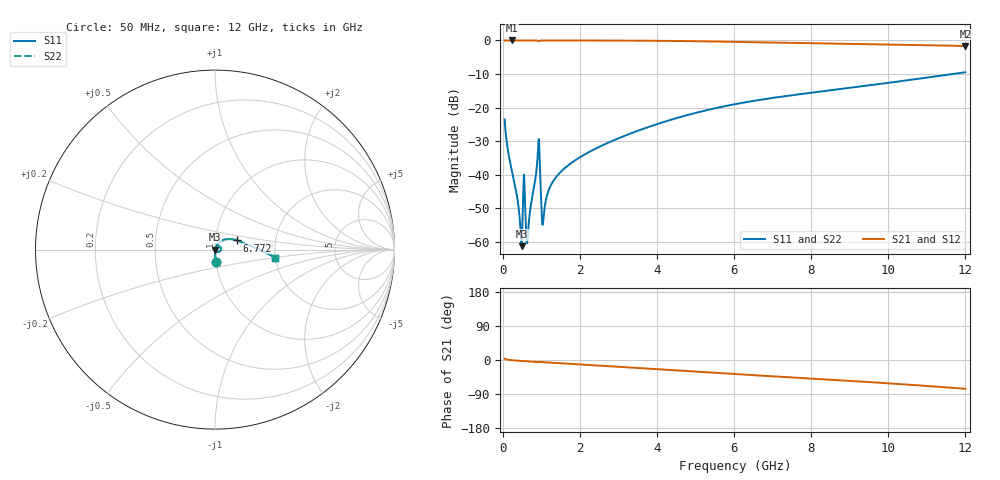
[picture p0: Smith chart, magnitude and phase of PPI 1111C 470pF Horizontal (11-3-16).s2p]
# MHz S MA R 50
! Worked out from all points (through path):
!   1601 points, 50 MHz to 12 GHz, reference 50 ohm
!   highest |S21| = 0.00 dB at 244.2 MHz (marker M1); lowest = -1.7 dB at 12 GHz (marker M2)
!   group delay of S21, straight-line fit = 17.5 ps
!   lowest |S11| = -61.3 dB at 490.7 MHz (marker M3), VSWR 1.00, Z = 50.1 - j0.00423 ohm
!   |S11| at or under -10 dB: start of sweep to 11.67 GHz
!   |S22| runs from -61.3 to -9.5 dB; largest |S21 - S12| = 0
!   S11 on the Smith chart (normalised r, x): 50 MHz: 1.00, -0.13; 6.772 GHz: 1.27, +0.13; 12 GHz: 1.98, -0.20
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50  0.06664 -86.2  0.9975 3.6  0.9975 3.6  0.06664 -86.2
244.1875  0.01111 -88.4  0.9995 -0.7  0.9995 -0.7  0.01111 -88.4
371.1562  0.004795 -85.4  0.9994 -1.7  0.9994 -1.7  0.004795 -85.4
445.8438  0.002067 -74.4  0.9993 -2.3  0.9993 -2.3  0.002067 -74.4
468.25  0.001279 -58.9  0.9993 -2.4  0.9993 -2.4  0.001279 -58.9
490.6562  0.0008631 -2.8  0.9991 -2.6  0.9991 -2.6  0.0008631 -2.8
565.3438  0.006683 -45.5  0.995 -2.7  0.995 -2.7  0.006683 -45.5
632.5625  0.0009554 9.8  0.999 -3.4  0.999 -3.4  0.0009554 9.8
662.4375  0.001539 52.9  0.9991 -3.6  0.9991 -3.6  0.001539 52.9
908.9062  0.01957 60.9  0.9921 -5.9  0.9921 -5.9  0.01957 60.9
946.25  0.02812 -24.0  0.9734 -4.5  0.9734 -4.5  0.02812 -24.0
1020.938  0.002078 -19.5  0.9979 -5.4  0.9979 -5.4  0.002078 -19.5
1058.281  0.002292 45.7  0.9985 -5.7  0.9985 -5.7  0.002292 45.7
1177.781  0.005566 72.6  0.9989 -6.6  0.9989 -6.6  0.005566 72.6
1334.625  0.008427 75.5  0.9989 -7.6  0.9989 -7.6  0.008427 75.5
2044.156  0.01882 73.3  0.9981 -11.9  0.9981 -11.9  0.01882 73.3
4038.312  0.0576 55.1  0.9876 -24.4  0.9876 -24.4  0.0576 55.1
6025  0.1124 30.8  0.9519 -37.1  0.9519 -37.1  0.1124 30.8
6771.875  0.1331 22.6  0.9346 -41.6  0.9346 -41.6  0.1331 22.6
8019.156  0.1669 12.1  0.9081 -49.0  0.9081 -49.0  0.1669 12.1
10013.31  0.234 1.6  0.8716 -61.6  0.8716 -61.6  0.234 1.6
12000  0.3359 -7.8  0.8248 -76.0  0.8248 -76.0  0.3359 -7.8
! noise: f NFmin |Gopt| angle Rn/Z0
50  0.0003424  0.8552  0.313  0.0005052
1372  0.003686  0.6692  7.244  0.002133
2701  0.008532  0.7139  14.18  0.005797
4031  0.01971  0.8081  21.06  0.02067
5360  0.03786  0.8658  27.77  0.05714
6682  0.0587  0.8933  34.23  0.1096
8012  0.07707  0.905  40.5  0.1566
9341  0.0917  0.9098  46.51  0.1887
1.067e+04  0.1043  0.9125  52.25  0.2117
1.2e+04  0.1165  0.9153  57.73  0.2326
